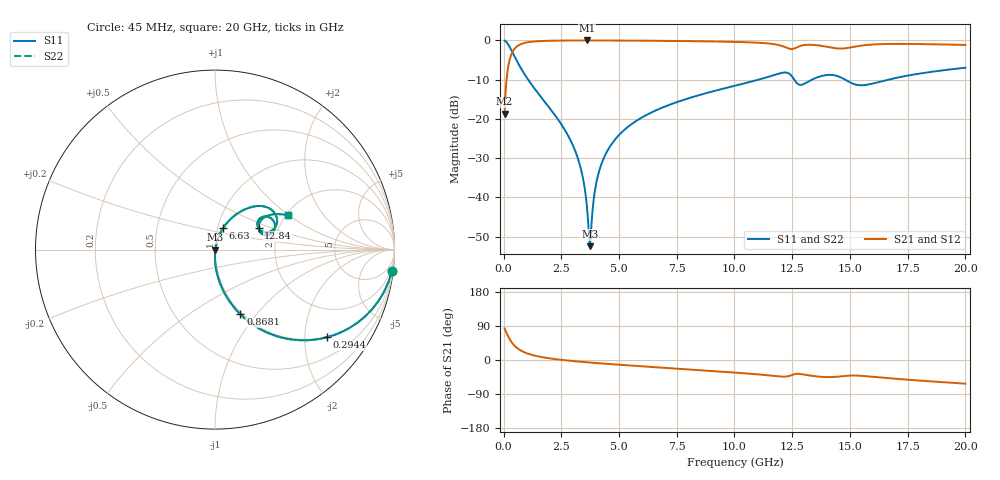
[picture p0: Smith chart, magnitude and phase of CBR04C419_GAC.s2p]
! S-parameter model data by Modelithics Inc.  support@modelithics.com 813-866-6335  Tampa FL USA
! S-Parameter data specifications:
! Substrate: 20-mil Rogers 4350B, substrate thickness, H=0.508mm, Dielectric constant, Er=3.75
! PCB Mounting Pad Footprint: Pad width, PadW=0.52mm , Pad length, PadL=0.52mm , Pad gap, PadG (edge-to-edge)=0.28mm , Reference planes=1.32mm apart
#  GHz  S  MA  R 50
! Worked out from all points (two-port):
!   801 points, 45 MHz to 20 GHz, reference 50 ohm
!   highest |S21| = -0.02 dB at 3.612 GHz (marker M1); lowest = -18.7 dB at 45 MHz (marker M2)
!   |S21| within 3 dB of the highest: 381.1 MHz to end of sweep
!   lowest |S11| = -52.5 dB at 3.737 GHz (marker M3), VSWR 1.00, Z = 50.2 - j0.0338 ohm
!   |S11| at or under -10 dB: 1.062 GHz to 11.05 GHz (9.988 GHz wide, 165 % of centre); 12.59 GHz to 13.36 GHz (769.4 MHz wide, 5.93 % of centre); 14.78 GHz to 16.67 GHz (1.889 GHz wide, 12 % of centre)
!   |S22| runs from -52.5 to -0.1 dB; largest |S21 - S12| = 0
!   S11 on the Smith chart (normalised r, x): 45 MHz: 1, -17; 294.4 MHz: 0.98, -2.57; 868.1 MHz: 0.98, -0.83; 6.63 GHz: 1.06, +0.26; 12.84 GHz: 1.58, +0.41; 20 GHz: 2.05, +0.98
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0.045  0.9932 -6.7  0.116 83.3  0.116 83.3  0.9932 -6.7
0.194662  0.892 -27.2  0.4518 62.8  0.4518 62.8  0.892 -27.2
0.294438  0.7926 -38.1  0.6093 51.9  0.6093 51.9  0.7926 -38.1
0.543875  0.5696 -56.2  0.8211 33.8  0.8211 33.8  0.5696 -56.2
0.868144  0.387 -68.6  0.9209 21.2  0.9209 21.2  0.387 -68.6
2.689037  0.06936 -89.2  0.9955 -0.8  0.9955 -0.8  0.06936 -89.2
3.387462  0.02064 -88.6  0.9974 -4.9  0.9974 -4.9  0.02064 -88.6
3.611956  0.007511 -77.9  0.9975 -6.1  0.9975 -6.1  0.007511 -77.9
3.736675  0.002381 -8.1  0.9975 -6.7  0.9975 -6.7  0.002381 -8.1
4.060944  0.01754 73.6  0.9972 -8.3  0.9972 -8.3  0.01754 73.6
4.509931  0.03973 75.9  0.9964 -10.3  0.9964 -10.3  0.03973 75.9
5.333075  0.07671 73.9  0.994 -13.9  0.994 -13.9  0.07671 73.9
6.63015  0.1294 69.2  0.988 -19.3  0.988 -19.3  0.1294 69.2
6.704981  0.1323 68.9  0.9875 -19.6  0.9875 -19.6  0.1323 68.9
10.0225  0.2644 55.0  0.956 -33.2  0.956 -33.2  0.2644 55.0
12.16766  0.3897 31.4  0.8265 -43.9  0.8265 -43.9  0.3897 31.4
12.84114  0.2706 26.4  0.8483 -36.9  0.8483 -36.9  0.2706 26.4
13.36496  0.3171 34.7  0.8771 -41.8  0.8771 -41.8  0.3171 34.7
14.18811  0.363 23.7  0.8095 -45.1  0.8095 -45.1  0.363 23.7
14.93642  0.2986 15.5  0.8036 -41.1  0.8036 -41.1  0.2986 15.5
16.68248  0.3167 33.1  0.9002 -48.1  0.9002 -48.1  0.3167 33.1
20  0.4481 25.1  0.8743 -62.4  0.8743 -62.4  0.4481 25.1
